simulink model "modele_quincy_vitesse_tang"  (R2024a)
settings: Solver=VariableStepAuto  StartTime=0.0  StopTime=1.8  RelTol=1e-3
libraries: fl_lib x7, nesl_utility x4, batteryecm_lib x1

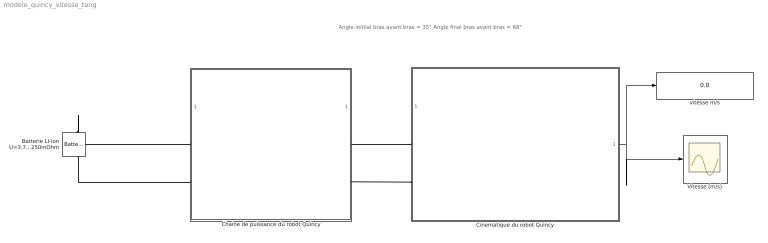
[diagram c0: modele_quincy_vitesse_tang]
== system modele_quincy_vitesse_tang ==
  note: Angle initilal bras avant bras = 35° Angle final bras avant bras = 68°
  Batterie LI-ion U=3.7V C=2.6A.h R=250mOhm : batteryecm_lib/Battery  Vnom=3.7 V  prm_dir=simscape.enum.battery.prm_dir.disabled  R1_dis=2 Ohm  R1_ch=2 Ohm  R1=0.25 Ohm  prm_AH=1  AH=50 hr*A  V1=11.5 V  AH1=25 hr*A  prm_R2=1  R2=2000 Ohm  Tmeas=298.15 K  charge_measurement_port=simscape.enum.battery.enable.no  prm_dyn=simscape.enum.battery.prm_dyn.off  Rp1=0.005 Ohm  tau1=30 s  Rp2=0.005 Ohm  tau2=30 s  Rp3=0.005 Ohm  tau3=30 s  Rp4=0.005 Ohm  tau4=30 s  Rp5=0.005 Ohm  tau5=30 s  prm_fade=1  N_fade=100  AH_fade=45 hr*A  R1_fade=2.02 Ohm  R1_ch_fade=2.02 Ohm  V1_fade=10.35 V  prm_age=simscape.enum.battery.prm_age.disabled  prm_age_OCV=simscape.enum.battery.prm_age_OCV.OCV  OCV_age=0.9  SOC_age=60  Tmeas_age=298.15 K  delta_time_age_vec=[0] d  temperature_age_vec=[273] K  OCV_scaling_age=2.2134e6  OCV_offset_age=1.632e6  temp_exp_age=0.515833569 V  t_exp_age=0.75  Vnom_T2=12 V  R1_T2=2.2 Ohm  R1_T2_dis=2.2 Ohm  R1_T2_ch=2.2 Ohm  V1_T2=11.4 V  R2_T2=2200 Ohm  Rp1_T2=0.005 Ohm  tau1_T2=30 s  Rp2_T2=0.005 Ohm  tau2_T2=30 s  Rp3_T2=0.005 Ohm  tau3_T2=30 s  Rp4_T2=0.005 Ohm  tau4_T2=30 s  Rp5_T2=0.005 Ohm  tau5_T2=30 s  Tmeas2=273.15 K  thermal_port=simscape.enum.thermaleffects.omit  thermal_mass=30000 J/K  i_specify=off  i_priority=None  i=0 A  i_nominal_specify=off  i_nominal_value=1  i_nominal_unit=A  v_specify=off  v_priority=None  v=0 V  v_nominal_specify=off  v_nominal_value=1  v_nominal_unit=V  charge_specify=off  charge_priority=High  charge=50 hr*A  charge_nominal_specify=off  charge_nominal_value=1  charge_nominal_unit=hr*A  num_cycles_specify=off  num_cycles_priority=High  num_cycles=0  num_cycles_nominal_specify=off  num_cycles_nominal_value=1  num_cycles_nominal_unit=1  temperature_specify=off  temperature_priority=High  temperature=298.15 K  temperature_nominal_specify=off  temperature_nominal_value=1  temperature_nominal_unit=K
  Chaine de puissance du robot Quincy : Subsystem  mask{r=32}
      mask prompts: r "rapport de réduction (1/r)"
  Cinematique du robot Quincy : Subsystem  mask{e=0.11, L=0.11, alpha1=35, alpha2=68}
      mask prompts: e "Longueur bras (m)"; L "Longueur avant-bras (m)"; alpha1 "Angle initial (degrés)"; alpha2 "Angle final (degrés)"
  Vitesse (m/s) : Scope  NumInputPorts=2
  vitesse m/s : Display
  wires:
  Cinematique du robot Quincy/1(Out1) -> Vitesse (m/s)/1, vitesse m/s/1
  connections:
  Cinematique du robot Quincy/LConn1 -- Chaine de puissance du robot Quincy/RConn1
  Batterie LI-ion U=3.7V C=2.6A.h R=250mOhm/LConn1 -- Chaine de puissance du robot Quincy/LConn1
  Batterie LI-ion U=3.7V C=2.6A.h R=250mOhm/RConn1 -- Chaine de puissance du robot Quincy/LConn2
  Cinematique du robot Quincy/LConn2 -- Chaine de puissance du robot Quincy/RConn2

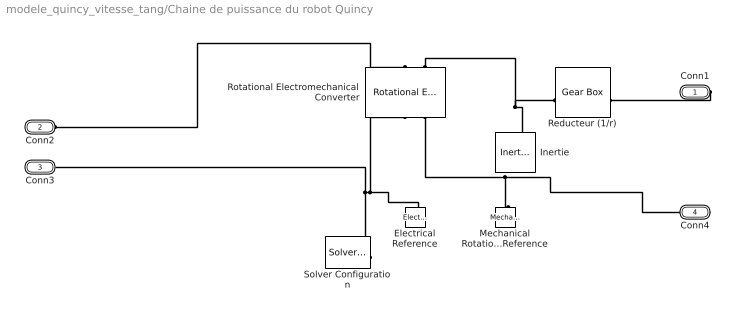
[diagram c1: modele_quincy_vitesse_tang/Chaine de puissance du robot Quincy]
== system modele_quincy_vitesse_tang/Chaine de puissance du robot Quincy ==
  Electrical Reference : fl_lib/Electrical/Electrical Elements/Electrical Reference
  Inertie : fl_lib/Mechanical/Rotational Elements/Inertia  inertia=0.2 kg*m^2  num_ports=foundation.enum.numPorts2.one  w_specify=off  w_priority=High  w=0 rad/s  w_nominal_specify=off  w_nominal_value=1  w_nominal_unit=rad/s  t_specify=off  t_priority=None  t=0 N*m  t_nominal_specify=off  t_nominal_value=1  t_nominal_unit=N*m
  Mechanical Rotational Reference : fl_lib/Mechanical/Rotational Elements/Mechanical Rotational Reference
  Reducteur (1/r) : fl_lib/Mechanical/Mechanisms/Gear Box  ratio=r  t_in_specify=off  t_in_priority=None  t_in=0 N*m  t_in_nominal_specify=off  t_in_nominal_value=1  t_in_nominal_unit=N*m  t_out_specify=off  t_out_priority=None  t_out=0 N*m  t_out_nominal_specify=off  t_out_nominal_value=1  t_out_nominal_unit=N*m
  Rotational Electromechanical Converter : fl_lib/Electrical/Electrical Elements/Rotational Electromechanical Converter  K=0.95 V/(rad/s)  i_specify=off  i_priority=None  i=0 A  i_nominal_specify=off  i_nominal_value=1  i_nominal_unit=A  v_specify=off  v_priority=None  v=0 V  v_nominal_specify=off  v_nominal_value=1  v_nominal_unit=V  t_specify=off  t_priority=None  t=0 N*m  t_nominal_specify=off  t_nominal_value=1  t_nominal_unit=N*m  w_specify=off  w_priority=None  w=0 rad/s  w_nominal_specify=off  w_nominal_value=1  w_nominal_unit=rad/s
  Solver Configuration : nesl_utility/Solver Configuration  PhysicalDomain=network_engine_domain  SubClassName=solver  LeftPortType=input  RightPortType=generic  Tones=[]  Harmonics=[]  SimulateNoise=off  Profile=off  UseLocalSampling=off  EnableSwitchedLinearOptims=on  FrequencyDomain=off  UseCCode=off  RelTol=0.001  AbsTol=1e-06  MinStep=1e-09  ToWorkspace=off  RevertToSquareIcSolve=off  NumHomotopyIterations=100  PhasorMode=off  PhasorModeNumHarmonics=1  ConsistencySolver=NEWTON_FTOL  IndexReductionMethod=DerivativeReplacement  DoDC=off  ResidualTolerance=1e-09  ConsistencyTolSource=GLOBAL  ConsistencyAbsTol=0.001  ConsistencyRelTol=0.001  ConsistencyTolFactor=0.001  UseLocalSolver=off  LocalSolverChoice=NE_BACKWARD_EULER_ADVANCER  ResolveIndetEquations=on  FunctionEvalNumThread=1  LocalSolverSampleTime=0.001  DoFixedCost=off  MaxNonlinIter=3  MaxModeIter=2  ComputeImpulses=off  ImpulseIterations=2  LinearAlgebra=Sparse  LinearAlgebraNumThread=0  EquationFormulation=NE_TIME_EF  DelaysMemoryBudget=1024  AutomaticFiltering=on  FilteringTimeConstant=0.001  PartitionStorageMethod=AS_NEEDED  PartitionMemoryBudget=1024  PartitionMethod=FAST  MultibodyUseLocalSolver=off  MultibodyLocalSolverChoice=ODE1  MultibodyLocalSolverSampleTime=0.001
  Conn1 : PMIOPort  Side=Right
  Conn2 : PMIOPort  Port=2  Side=Left
  Conn3 : PMIOPort  Port=3  Side=Left
  Conn4 : PMIOPort  Port=4  Side=Right
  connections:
  Conn2/RConn1 -- Rotational Electromechanical Converter/LConn1
  Solver Configuration/RConn1 -- Conn3/RConn1 -- Electrical Reference/LConn1 -- Rotational Electromechanical Converter/RConn1
  Rotational Electromechanical Converter/LConn2 -- Inertie/LConn1 -- Reducteur (1/r)/LConn1
  Rotational Electromechanical Converter/RConn2 -- Conn4/RConn1 -- Mechanical Rotational Reference/LConn1
  Conn1/RConn1 -- Reducteur (1/r)/RConn1

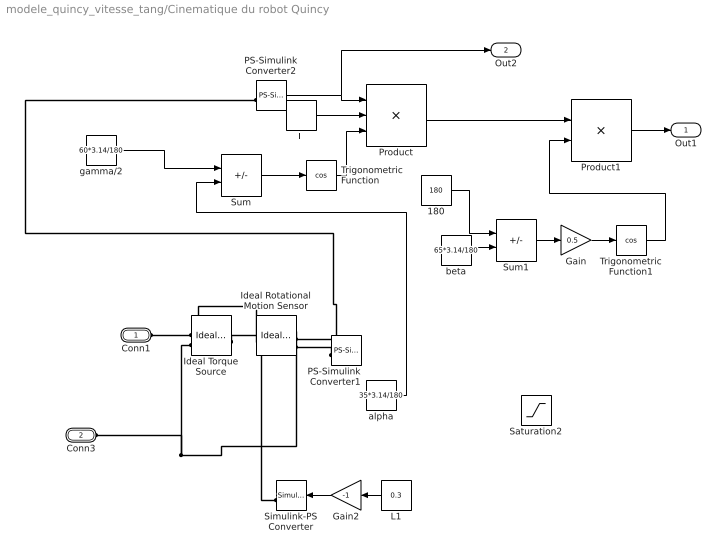
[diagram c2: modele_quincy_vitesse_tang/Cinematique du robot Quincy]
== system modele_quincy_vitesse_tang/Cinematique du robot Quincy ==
  180 : Constant  Value=180
  Gain : Gain  Gain=0.5
  Gain2 : Gain  Gain=-1
  Ideal Rotational Motion Sensor : fl_lib/Mechanical/Mechanical Sensors/Ideal Rotational Motion Sensor  reference=foundation.enum.MeasurementReference.difference  acceleration_port=false  velocity_port=true  position_port=true  wrap_angle=false  offset=(35*3.14)/180 rad
  Ideal Torque Source : fl_lib/Mechanical/Mechanical Sources/Ideal Torque Source
  L : Constant  Value=L
  L1 : Constant  Value=0.3
  PS-Simulink Converter1 : nesl_utility/PS-Simulink Converter  PhysicalDomain=network_engine_domain  SubClassName=ps_output  LeftPortType=input  RightPortType=output  PseudoPeriodic=off  Frequencies=[]  VectorFormat=1-D array  Unit=rad  AffineConversion=off
  PS-Simulink Converter2 : nesl_utility/PS-Simulink Converter  PhysicalDomain=network_engine_domain  SubClassName=ps_output  LeftPortType=input  RightPortType=output  PseudoPeriodic=off  Frequencies=[]  VectorFormat=1-D array  Unit=rad/s  AffineConversion=off
  Product : Product  Inputs=3
  Product1 : Product  Inputs=*/
  Saturation2 : Saturate  UpperLimit=(alpha2*3.14)/180  LowerLimit=(alpha1*3.14)/180
  Simulink-PS Converter : nesl_utility/Simulink-PS Converter  PhysicalDomain=network_engine_domain  SubClassName=ps_input  LeftPortType=input  RightPortType=output  PseudoPeriodic=off  Frequencies=[]  NoiseDistribution=none  NoiseParameters=[]  Unit=N*m  AffineConversion=off  FilteringAndDerivatives=provide  SimscapeFilterOrder=1  InputFilterTimeConstant=0.001  UdotUserProvided=0
  Sum : Sum  Inputs=+-
  Sum1 : Sum  Inputs=+-
  Trigonometric Function : Trigonometry  Operator=cos
  Trigonometric Function1 : Trigonometry  Operator=cos
  alpha : Constant  Value=35*3.14/180
  beta : Constant  Value=65*3.14/180
  gamma/2 : Constant  Value=60*3.14/180
  Conn1 : PMIOPort  Side=Left
  Conn3 : PMIOPort  Port=2  Side=Left
  Out1 : Outport
  Out2 : Outport  Port=2
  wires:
  L1/1 -> Gain2/1
  Gain2/1 -> Simulink-PS Converter/1
  PS-Simulink Converter2/1 -> Out2/1, Product/1
  L/1 -> Product/2
  gamma/2/1 -> Sum/1
  Sum/1 -> Trigonometric Function/1
  Trigonometric Function/1 -> Product/3
  Product/1 -> Product1/1
  beta/1 -> Sum1/2
  180/1 -> Sum1/1
  Sum1/1 -> Gain/1
  Gain/1 -> Trigonometric Function1/1
  Trigonometric Function1/1 -> Product1/2
  Product1/1 -> Out1/1
  alpha/1 -> Sum/2
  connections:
  Ideal Torque Source/LConn1 -- Ideal Rotational Motion Sensor/LConn1 -- Conn1/RConn1
  Simulink-PS Converter/RConn1 -- Ideal Torque Source/RConn1
  Ideal Torque Source/RConn2 -- Conn3/RConn1 -- Ideal Rotational Motion Sensor/RConn1
  PS-Simulink Converter1/LConn1 -- Ideal Rotational Motion Sensor/RConn3
  PS-Simulink Converter2/LConn1 -- Ideal Rotational Motion Sensor/RConn2
